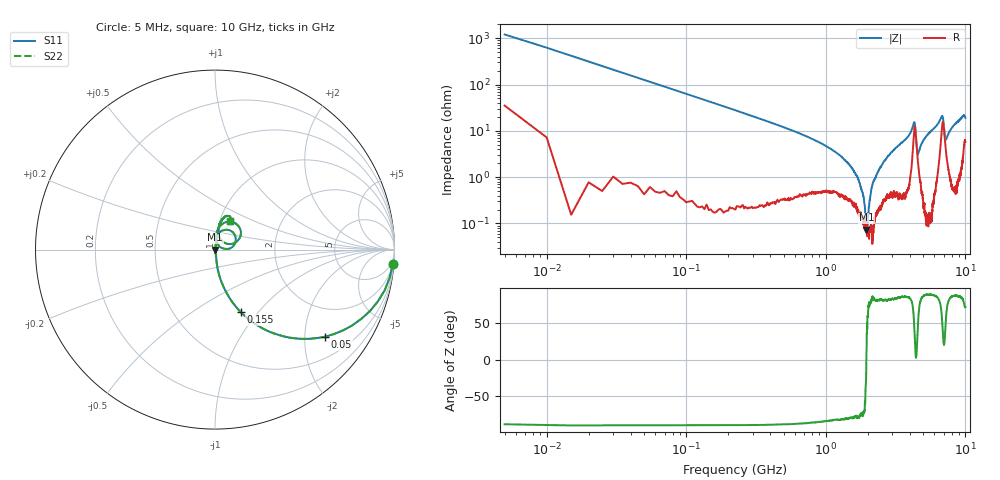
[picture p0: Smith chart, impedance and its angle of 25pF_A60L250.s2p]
! Amotech Co.,Ltd.
! http://www.amotech.co.kr/
! Part Number: A60L250
! These Parameters are Measured in Series Mode Connection
! Operation Temp=25[degC], DC Bias Voltage=0[V]
! Freq. Start=5[MHz] Stop=10[GHz], 2000[Steps]
! Date: Monday, July 14, 2020, 09:38:49
# GHZ S RI R 50.000000
!Freq.(Hz) S11(Real) S11(Imag) S21(Real) S21(Imag) S12(Real) S12(Imag) S22(Real) S22(Imag)
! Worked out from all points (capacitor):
!   2000 points, 5 MHz to 10 GHz, reference 50 ohm
!   read as one part in series: C = 25.2 pF near 55 MHz
!   lowest |Z| = 73.6 mohm at 1.955 GHz (marker M1)
!   series resonance near 1.952 GHz, so ESL is about 260 pH
!   S11 on the Smith chart (normalised r, x): 5 MHz: 2, -24; 50 MHz: 1.01, -2.52; 155 MHz: 1.00, -0.81; 10 GHz: 1.12, +0.36
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0.005  0.9908 -0.082  0.00919 0.082  0.00919 0.082  0.9908 -0.082
0.05  0.6129 -0.4854  0.3871 0.4854  0.3871 0.4854  0.6129 -0.4854
0.085  0.3556 -0.4754  0.6444 0.4754  0.6444 0.4754  0.3556 -0.4754
0.155  0.1425 -0.3474  0.8575 0.3474  0.8575 0.3474  0.1425 -0.3474
0.54  0.0152 -0.1072  0.9848 0.1072  0.9848 0.1072  0.0152 -0.1072
1.675  0.00238 -0.0101  0.9976 0.0101  0.9976 0.0101  0.00238 -0.0101
1.845  0.000974 -0.00419  0.999 0.00419  0.999 0.00419  0.000974 -0.00419
1.955  0.000724 0.000131  0.9993 -0.000131  0.9993 -0.000131  0.000724 0.000131
1.995  0.000577 0.000973  0.9994 -0.000973  0.9994 -0.000973  0.000577 0.000973
2.15  0.000525 0.00662  0.9995 -0.00662  0.9995 -0.00662  0.000525 0.00662
2.34  0.00203 0.0121  0.998 -0.0121  0.998 -0.0121  0.00203 0.0121
2.77  0.00482 0.0274  0.9952 -0.0274  0.9952 -0.0274  0.00482 0.0274
3.34  0.00613 0.0485  0.9939 -0.0485  0.9939 -0.0485  0.00613 0.0485
4.285  0.0961 0.0995  0.9039 -0.0995  0.9039 -0.0995  0.0961 0.0995
4.36  0.1101 0.0318  0.8899 -0.0318  0.8899 -0.0318  0.1101 0.0318
4.55  0.0238 0.0183  0.9762 -0.0183  0.9762 -0.0183  0.0238 0.0183
5.005  0.00613 0.0621  0.9939 -0.0621  0.9939 -0.0621  0.00613 0.0621
6.67  0.0803 0.1559  0.9197 -0.1559  0.9197 -0.1559  0.0803 0.1559
6.88  0.1445 0.0952  0.8555 -0.0952  0.8555 -0.0952  0.1445 0.0952
7.22  0.043 0.0449  0.957 -0.0449  0.957 -0.0449  0.043 0.0449
8.335  0.0227 0.1306  0.9773 -0.1306  0.9773 -0.1306  0.0227 0.1306
10  0.0821 0.1578  0.9179 -0.1578  0.9179 -0.1578  0.0821 0.1578
